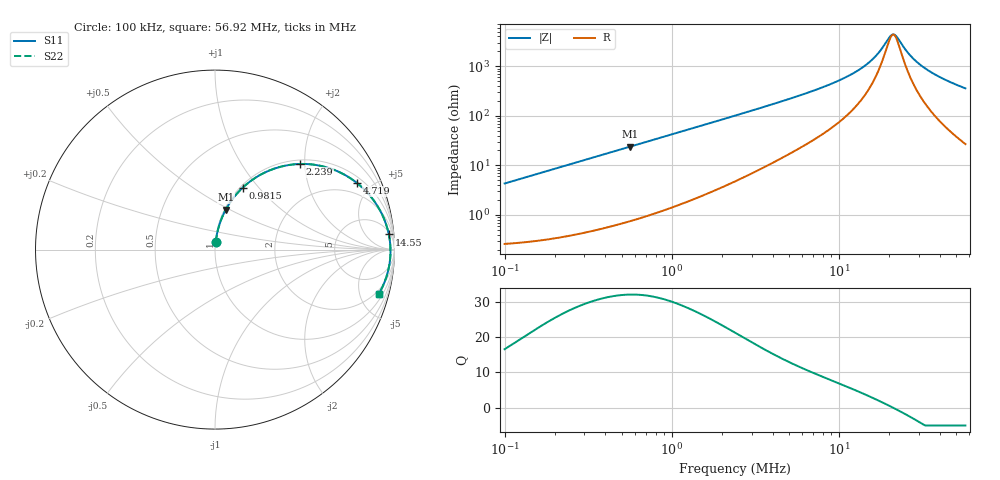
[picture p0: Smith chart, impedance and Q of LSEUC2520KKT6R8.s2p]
! LSEUC2520KKT6R8  S-PARAMETER MODEL  ( General Type )
! Model Generated by TAIYO YUDEN Corporation (http://www.ty-top.com)
! Version 1.0
! TAIYO YUDEN Control No. 211126
! Copyright(c) 2021 TAIYO YUDEN CO.,LTD. All Rights Reserved.
! Product Description (link to TY-COMPAS)
! https://ds.yuden.co.jp/TYCOMPAS/or/detail?pn=LSEUC2520KKT6R8M&u=M
! Products Name : Inductors
! Characteristics :
!  Inductance : 6.8 uH , SRF(min) : -Hz , DC Resistance(max) : 0.265 Ohm
!  Rated Current : Saturation :1200 mA , Temp Rise : 1300 mA (40 degC)
!  Case Size : 2.5 x 2.0 / 0.098 x 0.079 [mm/inch] , Thickness : 1 / 0.039 [mm/inch]
!  (Conditions: Temperature = 25 degC , DC Bias Current/Voltage = 0A / 0V)
! External Node Assignments :
!  1  o---GGG---o  2
! GND o---------o GND
! Frequency Range : 0.1MHz  -  56.923153MHz  [ 402 STEP ]
# MHz S RI R 50
! Freq[MHz].  S11 Real  S11 Imag  S21 Real  S21 Imag  S12 Real  S12 Imag  S22 Real  S22 Imag
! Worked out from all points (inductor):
!   401 points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, 100 kHz to 56.92 MHz, reference 50 ohm
!   read as one part in series: L = 6.84 uH near 103.2 kHz
!   highest Q = 32 at 563.4 kHz (marker M1), where L = 6.76 uH
!   self-resonance near 21.06 MHz
!   S11 on the Smith chart (normalised r, x): 100 kHz: 1.01, +0.09; 981.5 kHz: 1.03, +0.83; 2.239 MHz: 1.09, +1.89; 4.719 MHz: 1.30, +4.08; 14.55 MHz: 7, +21; 56.92 MHz: 1.54, -7.15
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0.1  0.00443 0.0427  0.9956 -0.0427  0.9956 -0.0427  0.00443 0.0427
0.289408  0.0192 0.1209  0.9808 -0.1209  0.9808 -0.1209  0.0192 0.1209
0.563399  0.0605 0.2233  0.9395 -0.2233  0.9395 -0.2233  0.0605 0.2233
0.837571  0.1195 0.3087  0.8805 -0.3087  0.8805 -0.3087  0.1195 0.3087
0.981531  0.1552 0.3458  0.8448 -0.3458  0.8448 -0.3458  0.1552 0.3458
1.436221  0.2761 0.4288  0.7239 -0.4288  0.7239 -0.4288  0.2761 0.4288
2.239193  0.4734 0.4771  0.5266 -0.4771  0.5266 -0.4771  0.4734 0.4771
2.424  0.5117 0.4767  0.4883 -0.4767  0.4883 -0.4767  0.5117 0.4767
3.276491  0.652 0.4486  0.348 -0.4486  0.348 -0.4486  0.652 0.4486
4.71887  0.7904 0.3717  0.2096 -0.3717  0.2096 -0.3717  0.7904 0.3717
6.904868  0.8864 0.2712  0.1136 -0.2712  0.1136 -0.2712  0.8864 0.2712
10.76529  0.9478 0.1563  0.0522 -0.1563  0.0522 -0.1563  0.9478 0.1563
14.5513  0.9685 0.0843  0.0315 -0.0843  0.0315 -0.0843  0.9685 0.0843
17.05234  0.9744 0.0479  0.0256 -0.0479  0.0256 -0.0479  0.9744 0.0479
19.98326  0.9774 0.0119  0.0226 -0.0119  0.0226 -0.0119  0.9774 0.0119
20.95709  0.9778 0.00115  0.0222 -0.00115  0.0222 -0.00115  0.9778 0.00115
21.97838  0.9778 -0.00964  0.0222 0.00964  0.0222 0.00964  0.9778 -0.00964
27.01111  0.9753 -0.057  0.0247 0.057  0.0247 0.057  0.9753 -0.057
29.70789  0.9723 -0.0794  0.0277 0.0794  0.0277 0.0794  0.9723 -0.0794
33.72699  0.9665 -0.11  0.0335 0.11  0.0335 0.11  0.9665 -0.11
42.78593  0.9488 -0.1703  0.0512 0.1703  0.0512 0.1703  0.9488 -0.1703
56.92315  0.9119 -0.2483  0.0881 0.2483  0.0881 0.2483  0.9119 -0.2483
